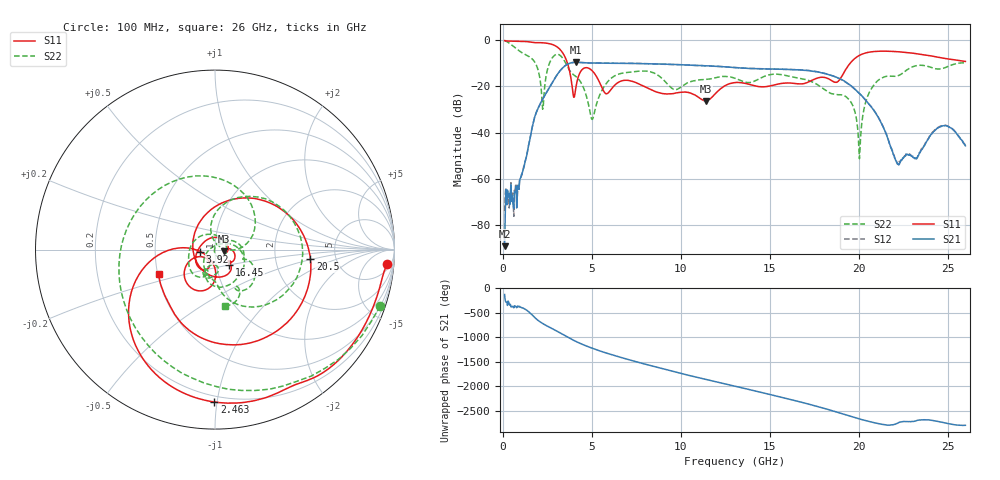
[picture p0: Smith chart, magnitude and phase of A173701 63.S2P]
!  2-Port S-parameters saved by WinCal
! VAR MeasName=S-Parameters (CALIBRATED_DATA) read from VNA (N5245A)
! VAR MeasDate=2017-6-7 10:32:37
! VAR NAME=A173701 63
! VAR FILENAME=A173701 63.S2P
! VAR DATE=2017-6-7 10:32:37
! VAR PHYS_PORTS=1,2
# Hz S DB R 50
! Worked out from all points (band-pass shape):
!   801 points, 100 MHz to 26 GHz, reference 50 ohm
!   highest |S21| = -9.68 dB at 4.114 GHz (marker M1); lowest = -89.0 dB at 100 MHz (marker M2)
!   |S21| within 3 dB of the highest: 3.292 GHz to 15.66 GHz (12.37 GHz wide, 131 % of centre); 15.68512 GHz to 15.7391 GHz (53.98 MHz wide, 0.344 % of centre)
!   lowest |S11| = -26.3 dB at 11.4 GHz (marker M3), VSWR 1.10, Z = 55 - j0.996 ohm
!   |S11| at or under -10 dB: 3.63 GHz to 19.53 GHz (15.9 GHz wide, 137 % of centre)
!   |S22| runs from -51.3 to -0.2 dB; largest |S21 - S12| = 0.0039
!   S11 on the Smith chart (normalised r, x): 100 MHz: 9, -20; 2.463 GHz: 0.16, -0.98; 3.92 GHz: 0.85, -0.02; 16.45 GHz: 1.15, -0.20; 20.5 GHz: 3.22, -0.48; 26 GHz: 0.51, -0.16
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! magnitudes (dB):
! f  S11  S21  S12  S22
! 100 MHz  -0.3  -89.0  -73.9  -0.2
! 909.4 MHz  -0.6  -64.4  -64.5  -4.7
! 2.237 GHz  -1.2  -25.6  -25.6  -29.9
! 2.463 GHz  -1.4  -22.6  -22.5  -14.3
! 3.046 GHz  -3.0  -15.1  -15.1  -6.2
! 3.92 GHz  -21.6  -9.8  -9.8  -14.7
! 4.114 GHz  -20.2  -9.7  -9.7  -15.8
! 4.438 GHz  -13.0  -9.8  -9.8  -19.1
! 5.021 GHz  -13.3  -10.0  -10.0  -34.3
! 6.251 GHz  -19.8  -10.1  -10.1  -15.7
! 8.744 GHz  -22.7  -10.4  -10.4  -15.4
! 11.4 GHz  -26.3  -11.2  -11.1  -17.0
! 13.05 GHz  -18.4  -11.9  -11.9  -16.6
! 16.45 GHz  -18.9  -12.9  -12.8  -16.3
! 17.39 GHz  -17.4  -13.5  -13.4  -18.2
! 19.46 GHz  -10.7  -19.2  -19.3  -25.8
! 20.04 GHz  -6.7  -23.1  -23.1  -51.3
! 20.5 GHz  -5.4  -26.9  -26.9  -24.5
! 21.69 GHz  -4.9  -43.8  -43.6  -15.6
! 22.21 GHz  -5.1  -53.5  -53.5  -15.5
! 24.7 GHz  -7.8  -37.2  -37.0  -12.4
! 26 GHz  -9.3  -45.7  -45.7  -10.0
